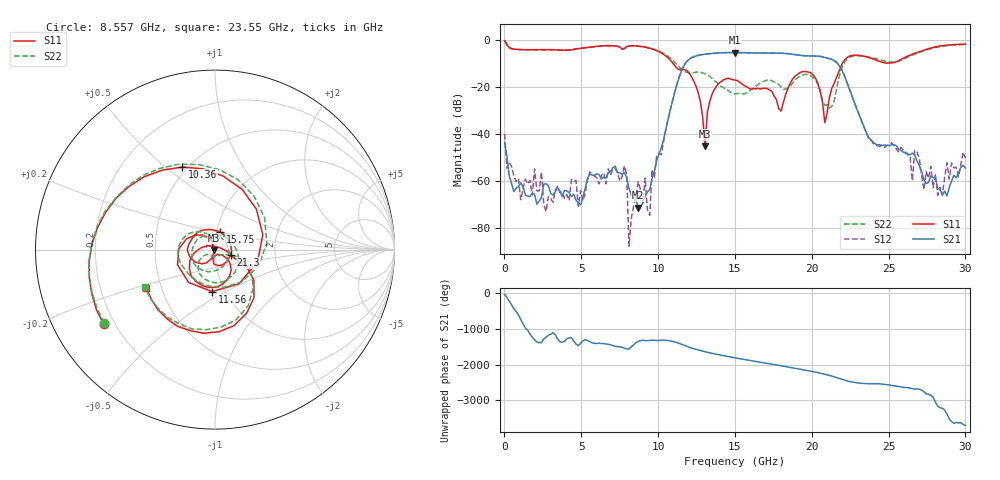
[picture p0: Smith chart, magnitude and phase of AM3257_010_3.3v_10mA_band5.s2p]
!Keysight Technologies,N5245B,MY58422270,A.16.20.02
!Date: Wednesday, June 18, 2025 23:00:42
!Correction: S11(C  2-Port  )
!S21(C  2-Port  )
!S12(C  2-Port  )
!S22(C  2-Port  )
!S2P File: Measurements: S11, S21, S12, S22:
# Hz S  dB  R 50
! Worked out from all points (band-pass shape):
!   201 points, 10 MHz to 30 GHz, reference 50 ohm
!   highest |S21| = -5.35 dB at 15.01 GHz (marker M1); lowest = -71.2 dB at 8.707 GHz (marker M2)
!   |S21| within 3 dB of the highest: 12 GHz to 21.33 GHz (9.331 GHz wide, 56 % of centre)
!   lowest |S11| = -45.2 dB at 13.06 GHz (marker M3), VSWR 1.01, Z = 49.5 - j0.262 ohm
!   |S11| at or under -10 dB: 10.98 GHz to 22 GHz (11.02 GHz wide, 66.8 % of centre)
!   |S22| runs from -28.9 to -0.2 dB; largest |S21 - S12| = 0.01
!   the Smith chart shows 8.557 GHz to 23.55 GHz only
!   S11 on the Smith chart (normalised r, x): 8.557 GHz: 0.16, -0.30; 10.36 GHz: 0.47, +0.57; 11.56 GHz: 0.87, -0.43; 15.75 GHz: 1.04, +0.20; 21.3 GHz: 1.19, -0.07; 23.55 GHz: 0.41, -0.22
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1e7  -0.30 -7.4  -43.47 -30.1  -39.97 41.4  -0.23 -7.7
6.098e8  -3.89 -167.3  -64.29 -63.7  -57.68 113.1  -3.92 -167.5
2.7091e9  -4.14 90.7  -61.01 -148.7  -72.83 -145.8  -4.11 90.9
5.1083e9  -3.46 -6.6  -66.63 109.6  -68.28 -51.4  -3.44 -4.9
8.55715e9  -2.54 -146.2  -67.80 52.8  -66.45 38.4  -2.61 -146.5
8.7071e9  -2.61 -153.2  -71.20 92.7  -60.17 57.4  -2.69 -153.7
9.45685e9  -3.52 169.7  -63.51 116.2  -74.44 -136.1  -3.49 168.8
1.005665e10  -4.94 134.1  -48.48 117.1  -48.12 108.8  -4.78 134.2
1.035655e10  -6.11 111.6  -42.25 127.3  -43.20 131.7  -5.73 112.9
1.155615e10  -12.60 -94.1  -12.65 4.8  -12.47 5.0  -12.63 -50.2
1.305565e10  -45.16 -151.4  -6.04 160.0  -6.04 159.9  -14.40 162.7
1.35055e10  -23.16 -117.9  -5.72 115.9  -5.71 115.9  -16.27 140.3
1.5005e10  -17.07 147.7  -5.35 -11.9  -5.35 -11.9  -22.93 76.3
1.575475e10  -19.85 72.9  -5.45 -69.5  -5.46 -69.5  -22.48 -0.6
1.83039e10  -23.14 -36.5  -5.74 101.2  -5.76 101.3  -20.88 73.1
2.01033e10  -15.01 -143.3  -6.84 -40.7  -6.85 -40.5  -15.97 -122.8
2.085305e10  -35.07 105.8  -7.45 -114.2  -7.44 -114.3  -27.81 -124.2
2.13029e10  -20.59 -18.3  -8.26 -165.4  -8.20 -165.0  -28.23 -62.0
2.355215e10  -7.17 -150.7  -39.34 -18.0  -39.33 -26.3  -7.07 -151.6
2.505165e10  -9.84 92.7  -44.89 -57.7  -44.50 -50.7  -9.37 101.6
2.82006e10  -2.75 -74.3  -63.07 65.7  -65.91 144.2  -3.04 -75.3
3e10  -1.80 -113.3  -54.37 -115.9  -50.07 -91.2  -1.94 -115.3
